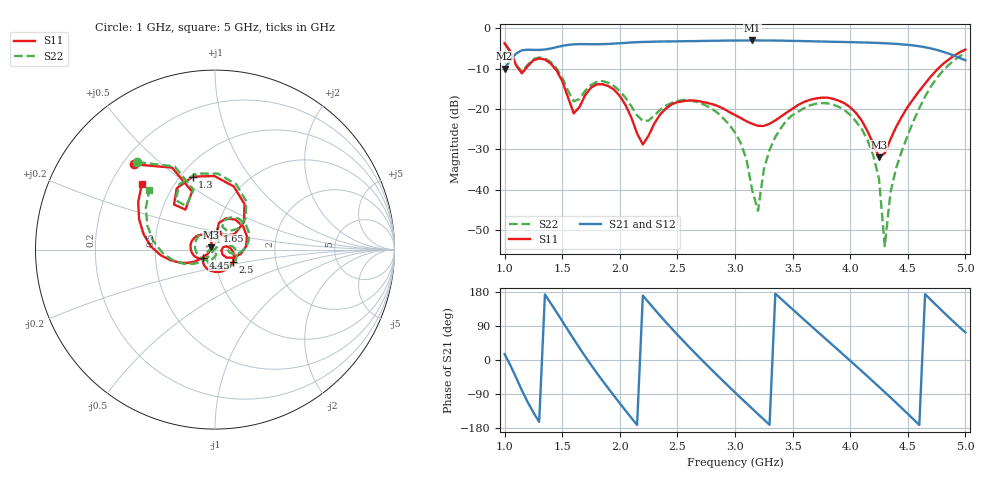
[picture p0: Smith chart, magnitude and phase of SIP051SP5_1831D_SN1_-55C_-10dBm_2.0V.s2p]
# GHz  S  dB  R  50
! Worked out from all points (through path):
!   81 points, 1 GHz to 5 GHz, reference 50 ohm
!   highest |S21| = -3.00 dB at 3.15 GHz (marker M1); lowest = -10.0 dB at 1 GHz (marker M2)
!   lowest |S11| = -31.9 dB at 4.25 GHz (marker M3), VSWR 1.05, Z = 47.8 + j1.22 ohm
!   |S11| at or under -10 dB: 1.121 GHz to 1.182 GHz (61.55 MHz wide, 5.34 % of centre); 1.438 GHz to 4.763 GHz (3.324 GHz wide, 107 % of centre)
!   |S22| runs from -54.0 to -3.7 dB; largest |S21 - S12| = 0.0027
!   S11 on the Smith chart (normalised r, x): 1 GHz: 0.25, +0.41; 1.3 GHz: 0.57, +0.57; 1.65 GHz: 1.00, +0.21; 2.5 GHz: 1.21, -0.17; 4.45 GHz: 0.87, -0.08; 5 GHz: 0.33, +0.34
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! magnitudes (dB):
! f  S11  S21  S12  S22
! 1 GHz  -3.7  -10.0  -10.0  -3.7
! 1.15 GHz  -11.1  -5.4  -5.4  -10.7
! 1.3 GHz  -7.4  -5.4  -5.4  -7.2
! 1.65 GHz  -19.5  -3.9  -3.9  -17.5
! 1.7 GHz  -16.5  -3.9  -3.9  -15.4
! 1.95 GHz  -15.2  -3.8  -3.8  -14.3
! 2.2 GHz  -28.8  -3.4  -3.4  -22.9
! 2.35 GHz  -21.3  -3.3  -3.3  -20.2
! 2.5 GHz  -18.3  -3.2  -3.2  -18.0
! 3 GHz  -21.5  -3.0  -3.0  -25.8
! 3.15 GHz  -23.7  -3.0  -3.0  -40.2
! 3.2 GHz  -24.2  -3.0  -3.0  -45.2
! 3.25 GHz  -24.2  -3.0  -3.0  -35.0
! 3.35 GHz  -22.8  -3.0  -3.0  -26.9
! 3.7 GHz  -17.4  -3.2  -3.2  -18.7
! 4.05 GHz  -21.0  -3.5  -3.5  -23.1
! 4.25 GHz  -31.9  -3.6  -3.6  -37.3
! 4.3 GHz  -30.9  -3.7  -3.7  -54.0
! 4.35 GHz  -27.5  -3.8  -3.8  -40.6
! 4.45 GHz  -21.8  -4.0  -4.0  -30.2
! 4.7 GHz  -11.9  -5.0  -5.0  -14.4
! 5 GHz  -5.3  -7.9  -7.9  -6.1
